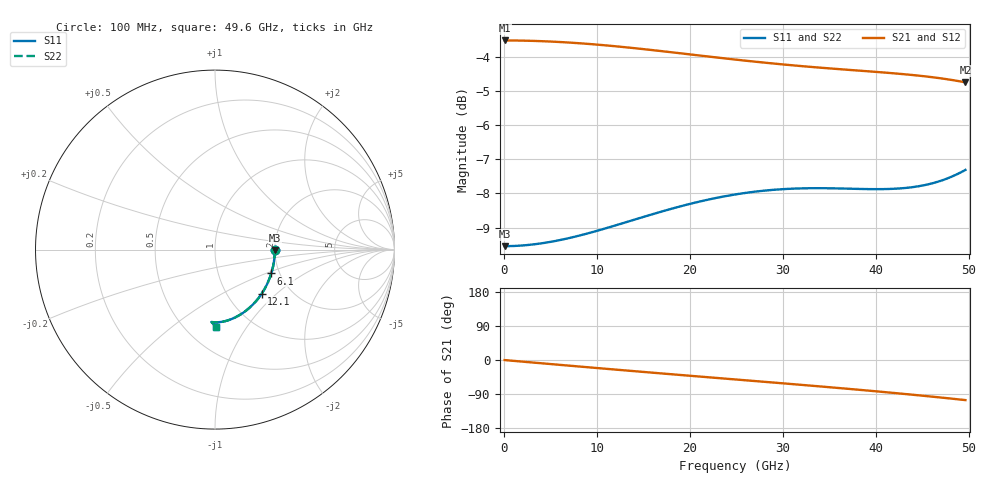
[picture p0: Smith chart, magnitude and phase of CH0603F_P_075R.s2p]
# GHz S RI R 75
! S-Parameters data
! Freq  reS11  imS11  reS21  imS21  reS12  imS12  reS22  imS22
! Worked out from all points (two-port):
!   100 points, 100 MHz to 49.6 GHz, reference 75 ohm
!   highest |S21| = -3.52 dB at 100 MHz (marker M1); lowest = -4.7 dB at 49.6 GHz (marker M2)
!   |S21| within 3 dB of the highest: start of sweep to end of sweep
!   lowest |S11| = -9.5 dB at 100 MHz (marker M3), VSWR 2.00, Z = 150 - j0.755 ohm
!   |S11| at or under -10 dB: nowhere
!   |S22| runs from -9.5 to -7.3 dB; largest |S21 - S12| = 0
!   S11 on the Smith chart (normalised r, x): 100 MHz: 2.00, -0.01; 6.1 GHz: 1.81, -0.54; 12.1 GHz: 1.43, -0.81; 49.6 GHz: 0.69, -0.73
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0.1  0.3333 -0.00224  0.6667 -0.00248  0.6667 -0.00248  0.3333 -0.00224
3.1  0.3281 -0.0689  0.6613 -0.0764  0.6613 -0.0764  0.3281 -0.0689
6.1  0.3133 -0.1331  0.6462 -0.1485  0.6462 -0.1485  0.3133 -0.1331
8.6  0.2944 -0.1832  0.6267 -0.2061  0.6267 -0.2061  0.2944 -0.1832
12.1  0.2597 -0.2461  0.5899 -0.2812  0.5899 -0.2812  0.2597 -0.2461
14.6  0.2305 -0.2849  0.5579 -0.3303  0.5579 -0.3303  0.2305 -0.2849
16.6  0.2053 -0.3118  0.5294 -0.3666  0.5294 -0.3666  0.2053 -0.3118
18.6  0.1792 -0.3351  0.4986 -0.4002  0.4986 -0.4002  0.1792 -0.3351
20.6  0.1528 -0.3546  0.4659 -0.4311  0.4659 -0.4311  0.1528 -0.3546
22.6  0.1266 -0.3705  0.4315 -0.4592  0.4315 -0.4592  0.1266 -0.3705
25.1  0.0952 -0.3857  0.3866 -0.4907  0.3866 -0.4907  0.0952 -0.3857
27.1  0.0716 -0.3942  0.3491 -0.513  0.3491 -0.513  0.0716 -0.3942
29.1  0.05 -0.4  0.3104 -0.5328  0.3104 -0.5328  0.05 -0.4
33.1  0.0142 -0.405  0.2293 -0.5649  0.2293 -0.5649  0.0142 -0.405
35.6  -0.00206 -0.405  0.176 -0.5797  0.176 -0.5797  -0.00206 -0.405
37.6  -0.0113 -0.4043  0.1318 -0.5884  0.1318 -0.5884  -0.0113 -0.4043
39.6  -0.017 -0.4036  0.0862 -0.594  0.0862 -0.594  -0.017 -0.4036
41.6  -0.0192 -0.4038  0.0392 -0.596  0.0392 -0.596  -0.0192 -0.4038
43.6  -0.0178 -0.4058  -0.00914 -0.5939  -0.00914 -0.5939  -0.0178 -0.4058
45.6  -0.0132 -0.4103  -0.0584 -0.5871  -0.0584 -0.5871  -0.0132 -0.4103
47.6  -0.00602 -0.4185  -0.1082 -0.575  -0.1082 -0.575  -0.00602 -0.4185
49.6  0.00303 -0.431  -0.1576 -0.557  -0.1576 -0.557  0.00303 -0.431
